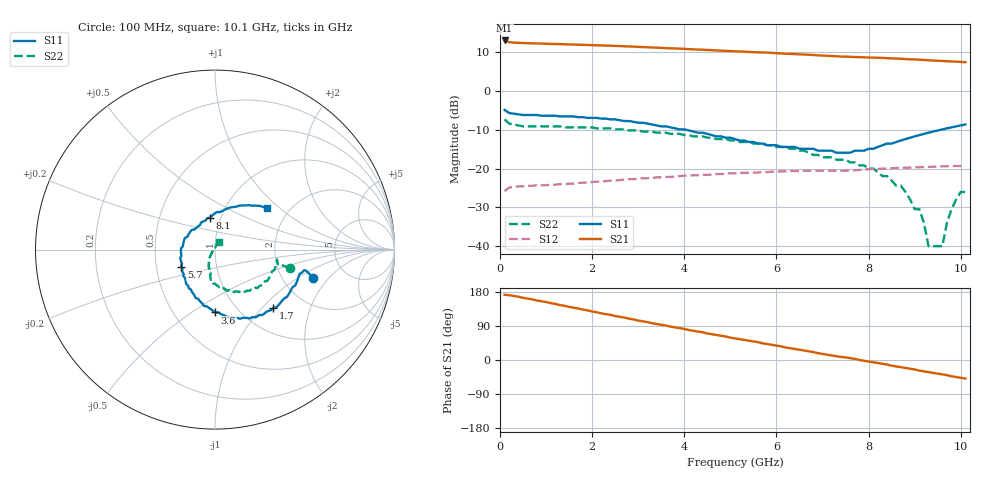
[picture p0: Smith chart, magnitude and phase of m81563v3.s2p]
!	MGA-81563 S PARAMETERS
!	Vd = 3 V LAST UPDATED 3-12-96
# ghz	s ma r	50
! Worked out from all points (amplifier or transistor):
!   101 points, 100 MHz to 10.1 GHz, reference 50 ohm
!   highest |S21| = 13.0 dB at 100 MHz (marker M1)
!   |S21| within 3 dB of that: start of sweep to 5.492 GHz
!   unconditionally stable (mu >= 1): start of sweep to end of sweep
!   at 1.7 GHz: K = 1.62, MAG = 13.2 dB, |S12| = -23.7 dB
!   at 5.1 GHz: K = 1.74, MAG = 10.7 dB, |S12| = -21.2 dB
!   at 10.1 GHz: K = 1.82, MAG = 8.1 dB, |S12| = -19.3 dB
!   lowest NFmin = 2.67 dB at 5.5 GHz
!   S11 on the Smith chart (normalised r, x): 100 MHz: 2.95, -1.37; 1.7 GHz: 1.41, -1.16; 3.6 GHz: 0.78, -0.62; 5.7 GHz: 0.67, -0.13; 8.1 GHz: 0.89, +0.33; 10.1 GHz: 1.54, +0.83
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0.1  0.57 -16.0  4.48 172.0  0.051 32.0  0.43 -14.0
0.2  0.52 -13.0  4.26 171.0  0.057 18.0  0.38 -13.0
1  0.48 -29.0  4.06 153.0  0.061 5.0  0.35 -15.0
1.3  0.47 -36.0  4.02 145.0  0.063 5.0  0.35 -19.0
1.7  0.46 -45.0  3.95 136.0  0.065 4.0  0.34 -26.0
1.8  0.46 -47.0  3.93 133.0  0.066 4.0  0.34 -27.0
2.5  0.43 -63.0  3.81 116.0  0.07 2.0  0.32 -39.0
3  0.39 -75.0  3.7 104.0  0.074 -1.0  0.31 -46.0
3.5  0.35 -87.0  3.59 93.0  0.077 -4.0  0.29 -53.0
3.6  0.35 -90.0  3.57 91.0  0.078 -5.0  0.29 -54.0
4.4  0.29 -112.0  3.4 73.0  0.083 -10.0  0.26 -66.0
5.1  0.24 -133.0  3.25 57.0  0.087 -17.0  0.23 -76.0
5.7  0.21 -153.0  3.14 44.0  0.09 -22.0  0.21 -84.0
6.8  0.18 159.0  2.91 21.0  0.094 -34.0  0.15 -100.0
8.1  0.18 99.0  2.69 -6.0  0.099 -44.0  0.1 -111.0
8.5  0.21 83.0  2.63 -15.0  0.101 -49.0  0.07 -118.0
9.1  0.27 63.0  2.53 -28.0  0.104 -55.0  0.03 -134.0
9.3  0.29 58.0  2.49 -32.0  0.105 -58.0  0.01 -153.0
9.6  0.32 50.0  2.44 -38.0  0.107 -61.0  0.01 87.0
9.8  0.34 46.0  2.4 -43.0  0.108 -63.0  0.03 73.0
10  0.36 41.0  2.37 -47.0  0.108 -66.0  0.05 66.0
10.1  0.37 39.0  2.35 -49.0  0.109 -67.0  0.05 64.0
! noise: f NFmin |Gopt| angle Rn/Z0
2  2.69  0.14  37  0.41
2.5  2.69  0.13  44  0.39
3.5  2.68  0.09  56  0.36
4.5  2.69  0.03  76  0.33
5.5  2.67  0.02  -135  0.32
6  2.69  0.05  -109  0.32
7  2.77  0.1  -78  0.36
8  2.77  0.16  -57  0.42
9  2.83  0.25  -41  0.54
10  2.8  0.35  -25  0.69
